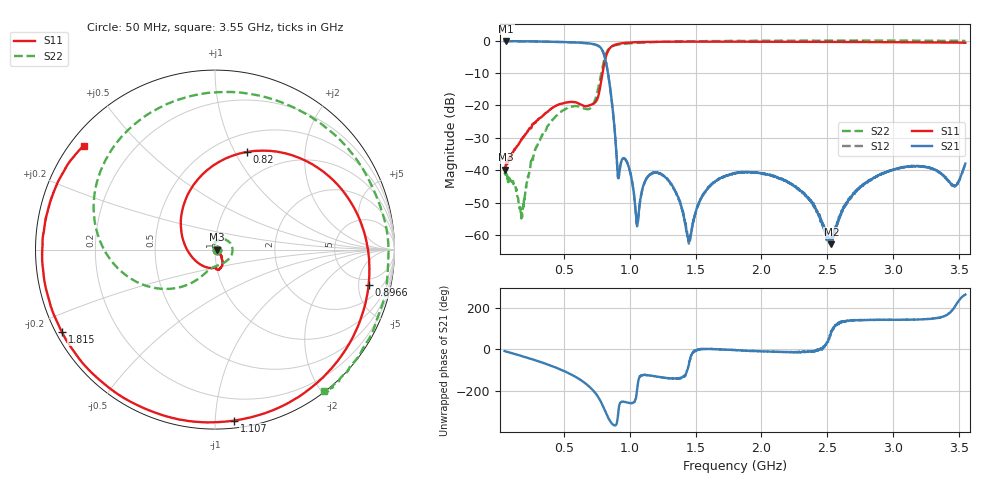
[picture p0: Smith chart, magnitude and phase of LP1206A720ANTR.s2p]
!Keysight Technologies,N5224B,MY57181629,A.13.20.12
!Date: Wednesday, January 30, 2019 10:36:28
!Correction: S11(Full 2 Port(1,2))
!S21(Full 2 Port(1,2))
!S12(Full 2 Port(1,2))
!S22(Full 2 Port(1,2))
!S2P File: Measurements: S11, S21, S12, S22:
!	LP1206 High Performance Low Pass Filters
!	P/N LP1206A0720ANTR 	30 Jan 2019
# Hz S  dB  R 50
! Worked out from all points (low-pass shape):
!   1601 points, 50 MHz to 3.55 GHz, reference 50 ohm
!   highest |S21| = -0.08 dB at 60.94 MHz (marker M1); lowest = -62.9 dB at 2.533 GHz (marker M2)
!   |S21| within 3 dB of the highest: start of sweep to 794 MHz
!   lowest |S11| = -39.8 dB at 56.56 MHz (marker M3), VSWR 1.02, Z = 51 - j0.111 ohm
!   |S11| at or under -10 dB: start of sweep to 793.4 MHz
!   |S22| runs from -54.9 to 0.1 dB; largest |S21 - S12| = 0.0037
!   S11 on the Smith chart (normalised r, x): 50 MHz: 1.02, -0.00; 820 MHz: 0.69, +1.12; 896.6 MHz: 3.83, -6.61; 1.107 GHz: 0.05, -1.12; 1.815 GHz: 0.02, -0.25; 3.55 GHz: 0.04, +0.35
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5e7  -39.27 -1.5  -0.10 -9.0  -0.11 -8.8  -41.23 -4.4
5.65625e7  -39.84 -6.1  -0.09 -10.4  -0.10 -10.4  -40.47 -2.3
6.09375e7  -38.17 -6.7  -0.08 -11.2  -0.10 -11.2  -42.03 -2.6
1.76875e8  -30.71 -36.5  -0.14 -32.5  -0.16 -32.5  -54.91 -124.8
3.3875e8  -23.23 -54.8  -0.23 -65.1  -0.24 -65.1  -28.90 94.1
6.340625e8  -19.79 -87.6  -0.60 -151.2  -0.61 -151.1  -20.60 -31.8
7.696875e8  -15.65 174.1  -1.75 119.9  -1.77 120.0  -13.01 -124.7
8.2e8  -4.85 72.0  -6.60 51.7  -6.61 51.8  -4.08 178.8
8.965625e8  -1.13 -13.0  -33.16 -4.6  -33.19 -4.2  -1.30 102.5
9.928125e8  -0.55 -56.0  -38.88 100.8  -39.06 100.9  -0.82 56.8
1.054062e9  -0.42 -72.6  -55.93 157.9  -56.81 151.1  -0.63 38.8
1.106562e9  -0.37 -83.7  -44.41 -124.5  -44.47 -123.6  -0.54 26.3
1.218125e9  -0.29 -101.6  -40.85 -133.2  -40.95 -132.8  -0.33 6.9
1.45e9  -0.27 -126.9  -60.58 -76.4  -62.74 -74.0  -0.16 -18.3
1.576875e9  -0.25 -136.8  -46.66 0.8  -46.59 1.6  -0.09 -27.0
1.8e9  -0.27 -150.7  -41.04 -4.2  -40.98 -4.1  -0.02 -37.5
1.815312e9  -0.28 -151.6  -40.78 -5.6  -40.76 -5.2  -0.02 -38.0
2.384062e9  -0.32 -177.6  -49.83 -10.5  -50.12 -7.1  0.07 -49.8
2.532812e9  -0.34 177.1  -62.89 82.5  -62.91 87.4  0.09 -51.0
2.705625e9  -0.37 171.1  -47.11 138.2  -47.10 140.6  0.11 -51.9
2.968125e9  -0.40 162.4  -40.32 142.6  -40.38 142.6  0.07 -52.6
3.55e9  -0.61 141.6  -37.96 -96.4  -37.99 -96.2  -0.05 -52.5
